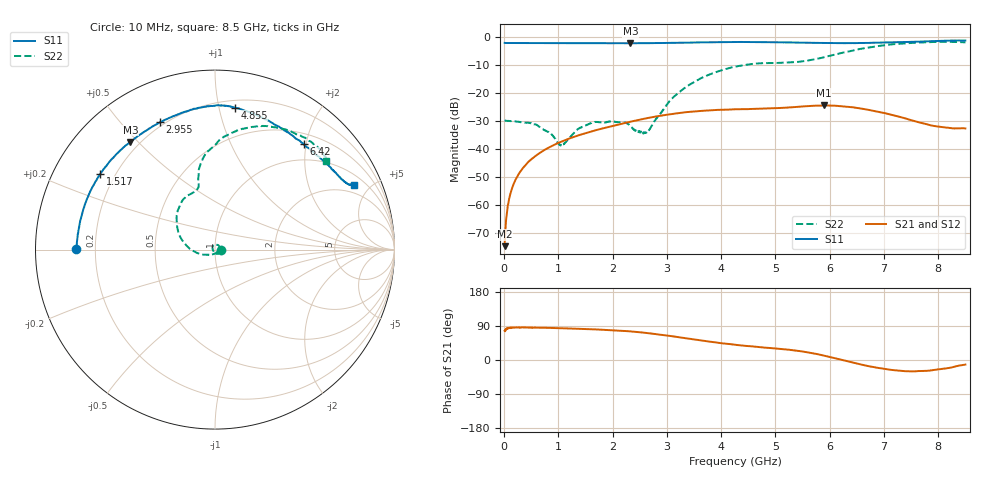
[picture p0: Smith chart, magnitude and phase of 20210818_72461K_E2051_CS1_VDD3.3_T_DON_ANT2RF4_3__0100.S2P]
!Agilent Technologies,E5071C,MY46417908,A.11.23
!Date: Wed Aug 18 14:32:57 2021
!Data & Calibration Information:
!Freq	S11:SOLT2(ON)	S21:SOLT2(ON)	S12:SOLT2(ON)	S22:SOLT2(ON)
!PortZ  Port1:50+j0  Port2:50+j0
!Above PortZ is port z conversion or system Z0 setting when saving the data.
!When reading, reference impedance value at option line is always used.
# Hz S dB R 50
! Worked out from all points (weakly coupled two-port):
!   1601 points, 10 MHz to 8.5 GHz, reference 50 ohm
!   highest |S21| = -24.55 dB at 5.889 GHz (marker M1); lowest = -74.8 dB at 10 MHz (marker M2)
!   lowest |S11| = -2.4 dB at 2.329 GHz (marker M3), VSWR 7.44, Z = 8.28 + j23.8 ohm
!   |S11| at or under -10 dB: nowhere
!   |S22| runs from -38.9 to -1.8 dB; largest |S21 - S12| = 0.00026
!   S11 on the Smith chart (normalised r, x): 10 MHz: 0.13, +0.00; 1.517 GHz: 0.14, +0.30; 2.955 GHz: 0.18, +0.64; 4.855 GHz: 0.25, +1.12; 6.42 GHz: 0.69, +1.96; 8.5 GHz: 1.51, +3.99
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1e7  -2.22 179.7  -74.81 77.1  -74.91 69.1  -29.82 -1.9
7.3675e7  -2.26 178.2  -59.99 83.1  -59.78 84.2  -30.09 -6.0
1.214312e8  -2.26 177.1  -55.77 85.1  -55.73 85.0  -30.16 -9.7
3.28375e8  -2.29 172.5  -47.36 86.2  -47.38 86.0  -30.58 -32.2
6.096062e8  -2.30 166.1  -42.17 85.4  -42.17 85.4  -31.59 -65.2
1.050025e9  -2.32 156.5  -37.53 83.8  -37.54 83.9  -38.62 -156.1
1.426769e9  -2.32 148.5  -34.90 82.0  -34.92 82.0  -32.30 117.4
1.516975e9  -2.32 146.5  -34.39 81.6  -34.38 81.7  -31.56 105.3
1.983925e9  -2.33 136.2  -31.94 78.6  -31.96 78.6  -30.26 48.4
2.328831e9  -2.35 128.1  -30.37 75.5  -30.37 75.5  -31.90 7.0
2.604756e9  -2.32 121.4  -29.21 71.7  -29.21 71.7  -34.16 -65.1
2.843538e9  -2.27 115.8  -28.36 67.5  -28.35 67.4  -28.24 -131.0
2.954969e9  -2.24 113.3  -28.01 65.5  -28.01 65.5  -25.56 -147.7
3.443144e9  -2.11 103.1  -26.79 55.5  -26.78 55.5  -16.83 177.1
4.255e9  -1.92 89.9  -25.93 40.3  -25.93 40.3  -10.72 136.8
4.854606e9  -1.95 82.1  -25.66 32.2  -25.66 32.2  -9.43 116.0
5.671769e9  -2.19 67.7  -24.71 18.4  -24.71 18.6  -8.25 103.9
5.889325e9  -2.24 62.6  -24.55 11.7  -24.55 11.7  -7.34 102.3
6.41995e9  -2.29 49.8  -25.20 -6.7  -25.22 -6.8  -4.99 92.2
7.088538e9  -2.04 35.3  -27.64 -25.2  -27.68 -25.4  -2.87 72.3
8.017131e9  -1.50 25.3  -32.13 -24.6  -32.10 -24.5  -1.86 45.5
8.5e9  -1.38 24.9  -32.77 -12.0  -32.83 -12.1  -2.02 38.4
